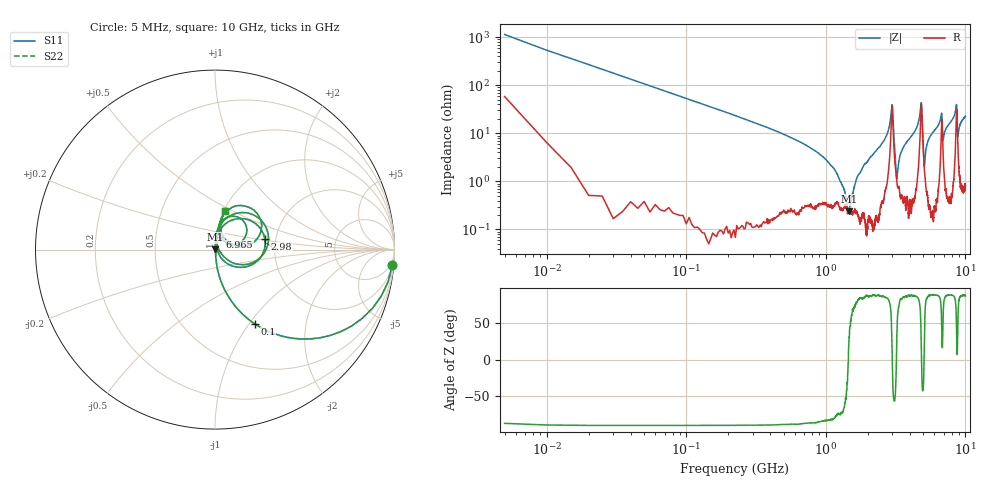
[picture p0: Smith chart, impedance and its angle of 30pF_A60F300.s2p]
! Amotech Co.,Ltd.
! http://www.amotech.co.kr/
! Part Number: A60F300
! These Parameters are Measured in Series Mode Connection
! Operation Temp=25[degC], DC Bias Voltage=0[V]
! Freq. Start=5[MHz] Stop=10[GHz], 2000[Steps]
! Date: Monday, July 20, 2020, 03:39:25
# GHZ S RI R 50.000000
!Freq.(Hz) S11(Real) S11(Imag) S21(Real) S21(Imag) S12(Real) S12(Imag) S22(Real) S22(Imag)
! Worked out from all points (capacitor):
!   2000 points, 5 MHz to 10 GHz, reference 50 ohm
!   read as one part in series: C = 29.7 pF near 55 MHz
!   lowest |Z| = 238 mohm at 1.465 GHz (marker M1)
!   series resonance near 1.451 GHz, so ESL is about 410 pH
!   S11 on the Smith chart (normalised r, x): 5 MHz: 2, -23; 100 MHz: 1.00, -1.07; 2.98 GHz: 1.75, +0.23; 6.965 GHz: 1.05, +0.15; 10 GHz: 1.02, +0.46
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0.005  0.988 -0.0865  0.012 0.0865  0.012 0.0865  0.988 -0.0865
0.1  0.2221 -0.4144  0.7779 0.4144  0.7779 0.4144  0.2221 -0.4144
0.345  0.0223 -0.1438  0.9777 0.1438  0.9777 0.1438  0.0223 -0.1438
1.16  0.00353 -0.017  0.9965 0.017  0.9965 0.017  0.00353 -0.017
1.465  0.00217 0.000977  0.9978 -0.000977  0.9978 -0.000977  0.00217 0.000977
1.675  0.00243 0.0119  0.9976 -0.0119  0.9976 -0.0119  0.00243 0.0119
2.72  0.0154 0.0873  0.9846 -0.0873  0.9846 -0.0873  0.0154 0.0873
2.98  0.2781 0.0597  0.7219 -0.0597  0.7219 -0.0597  0.2781 0.0597
3.205  0.0123 9.7e-05  0.9877 -9.7e-05  0.9877 -9.7e-05  0.0123 9.7e-05
3.34  0.00853 0.0254  0.9915 -0.0254  0.9915 -0.0254  0.00853 0.0254
4.55  0.0337 0.1424  0.9663 -0.1424  0.9663 -0.1424  0.0337 0.1424
4.805  0.2667 0.1519  0.7333 -0.1519  0.7333 -0.1519  0.2667 0.1519
4.885  0.1906 -0.0791  0.8094 0.0791  0.8094 0.0791  0.1906 -0.0791
5.005  0.0365 -0.0235  0.9635 0.0235  0.9635 0.0235  0.0365 -0.0235
5.09  0.0166 0.0118  0.9834 -0.0118  0.9834 -0.0118  0.0166 0.0118
5.41  0.00844 0.0704  0.9916 -0.0704  0.9916 -0.0704  0.00844 0.0704
6.67  0.084 0.1845  0.916 -0.1845  0.916 -0.1845  0.084 0.1845
6.965  0.0293 0.0721  0.9707 -0.0721  0.9707 -0.0721  0.0293 0.0721
8.335  0.0673 0.2174  0.9327 -0.2174  0.9327 -0.2174  0.0673 0.2174
8.63  0.25 0.1749  0.75 -0.1749  0.75 -0.1749  0.25 0.1749
8.835  0.0545 0.0601  0.9455 -0.0601  0.9455 -0.0601  0.0545 0.0601
10  0.0569 0.2128  0.9431 -0.2128  0.9431 -0.2128  0.0569 0.2128
